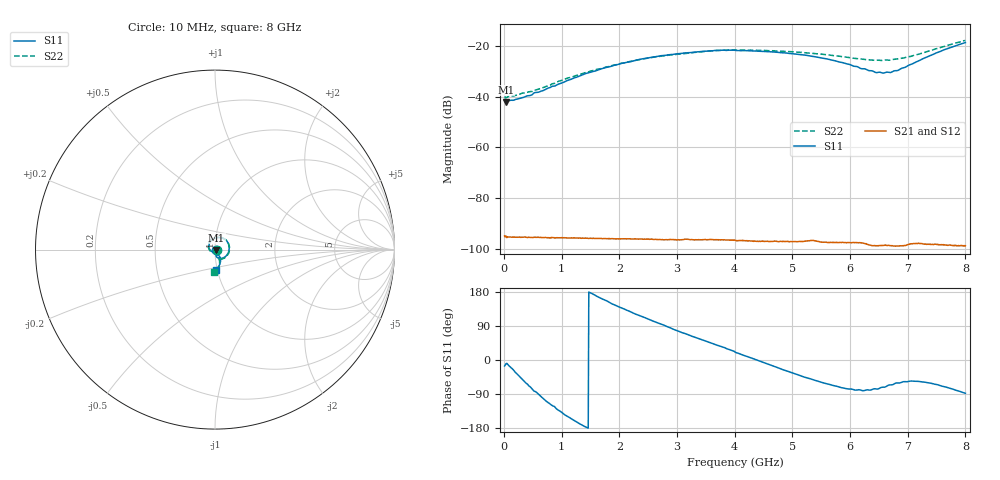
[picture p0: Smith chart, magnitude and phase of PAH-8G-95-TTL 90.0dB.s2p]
! MTS Systemtechnik GmbH
! S-Parameters
! Model: PAH-8G/95-TTL
! Attenuation Step: 90.0dB
! Rohde & Schwarz ZVB8 2Ports - Version 4.11 - 1145.1010k08 SN: 100119
! S2P File Measurements:
! S11 S21 S12 S22
# HZ  S  DB  R  50.00
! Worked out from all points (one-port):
!   800 points, 10 MHz to 8 GHz, reference 50 ohm
!   lowest |S11| = -42.2 dB at 30 MHz (marker M1), VSWR 1.02, Z = 50.8 - j0.147 ohm
!   |S11| at or under -10 dB: start of sweep to end of sweep
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1e7  -41.45 -15.7  -95.01 -2.9  -94.69 2.9  -39.99 -12.0
3e7  -42.20 -10.7  -94.99 -4.8  -95.44 -4.9  -40.58 -9.9
1.9e8  -41.26 -31.5  -95.48 -27.2  -95.46 -27.1  -39.62 -29.9
4.6e8  -39.57 -71.8  -95.60 -64.5  -95.57 -63.6  -38.03 -67.4
7.7e8  -36.63 -113.0  -95.70 -106.9  -95.63 -106.3  -35.71 -108.5
1.09e9  -33.74 -147.6  -95.76 -150.6  -95.83 -150.4  -32.78 -140.9
1.35e9  -31.56 -171.8  -95.82 173.9  -95.88 173.5  -31.04 -164.1
2.02e9  -27.03 138.4  -96.17 81.5  -96.15 82.0  -26.97 144.6
2.37e9  -25.25 116.0  -96.16 34.1  -96.19 34.2  -25.33 122.2
2.68e9  -24.10 96.7  -96.43 -9.0  -96.43 -8.3  -24.24 102.9
3.43e9  -22.24 53.9  -96.48 -110.4  -96.49 -110.0  -22.32 58.6
3.79e9  -21.74 34.2  -96.53 -160.1  -96.56 -159.7  -21.71 38.9
4.01e9  -21.85 20.2  -96.77 167.8  -96.71 168.8  -21.70 25.8
4.72e9  -22.52 -19.0  -97.04 71.4  -97.12 71.1  -22.03 -11.9
5.34e9  -24.15 -51.2  -96.76 -14.9  -96.87 -15.2  -22.96 -41.1
5.73e9  -25.85 -68.0  -97.53 -69.7  -97.53 -69.8  -23.90 -56.0
6.45e9  -30.56 -76.4  -98.82 -169.8  -98.86 -170.2  -25.69 -69.0
6.67e9  -30.48 -66.2  -98.69 161.7  -98.80 161.4  -25.70 -67.6
6.83e9  -29.73 -60.5  -98.91 142.4  -98.99 142.1  -25.18 -67.4
7.06e9  -27.30 -55.5  -98.04 112.1  -98.17 112.8  -24.14 -67.2
7.62e9  -21.66 -69.8  -98.39 29.3  -98.48 29.6  -20.34 -77.3
8e9  -18.74 -87.9  -98.86 -22.8  -98.87 -22.1  -17.90 -91.7
